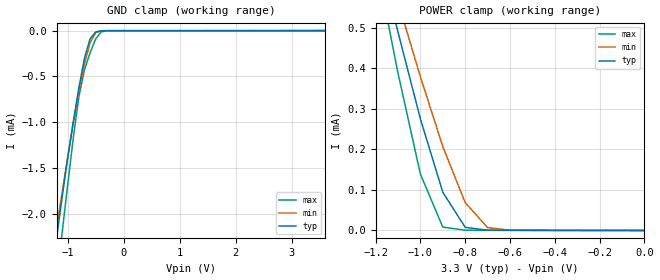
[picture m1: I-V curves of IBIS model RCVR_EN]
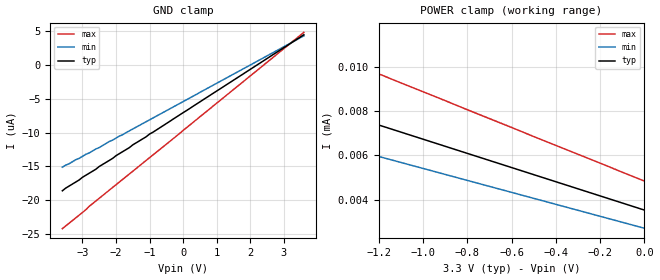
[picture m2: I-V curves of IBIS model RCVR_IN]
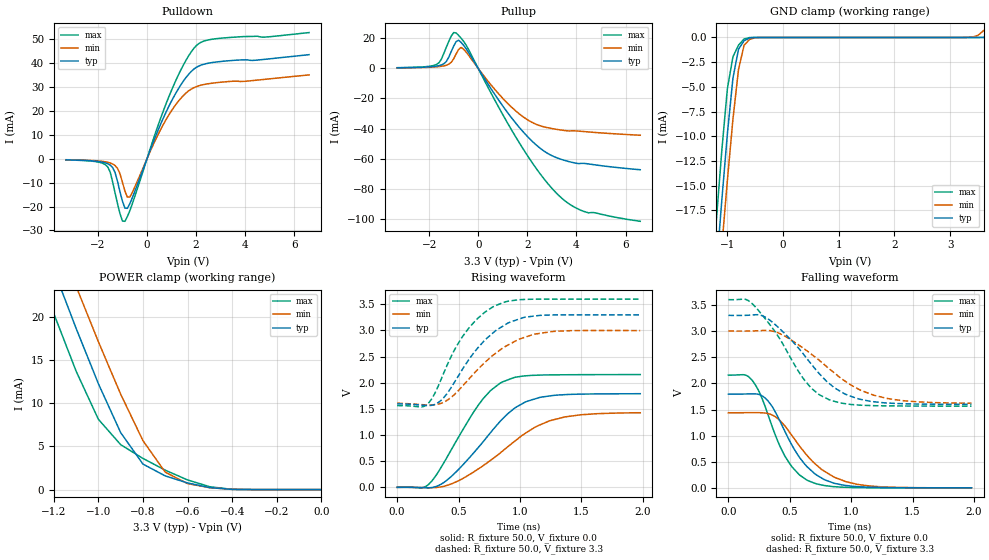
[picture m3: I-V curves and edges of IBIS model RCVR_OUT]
|   Texas Instruments Incorporated
|   Data Transmissions Products
|   IBIS Model for SN65MLVD2
|   8DRB SON Package
[IBIS Ver]   3.2
[Comment char]   |_char
[File name]   mlvd2.ibs
[File Rev]   1.0
[Date]   13Oct06
[Source]   File originated at Texas Instruments Incorporated.
   Data Transmission Products Group. All data based on
   Simulation Measurements.
[Notes]
[Disclaimer]
(C) Copyright Texas Instruments Incorporated 2006
   All rights reserved
  Texas Instruments Incorporated hereby grants the user of this IBIS
model a non-exclusive, nontransferable license to use this IBIS model
under the following terms.  Before using this IBIS model, the user
should read this license.  If the user does not accept these terms,
the IBIS model should be returned to Texas Instruments within 30 days.
  The user is granted this license only to use the IBIS model and
is not granted rights to sell, load, rent, lease or license the IBIS
model in whole or in part, or in modified form to anyone other than
user.  User may modify the IBIS model to suit its specific applications
but rights to derivative works and such modifications shall belong to
Texas Instruments.
  This IBIS model is provided on an "AS IS" basis and Texas Instruments
makes absolutely no warranty with respect to the information contained
herein.  TEXAS INSTRUMENTS DISCLAIMS AND CUSTOMER WAIVES ALL WARRANTIES,
EXPRESS OR IMPLIED, INCLUDING WARRANTIES OF MERCHANTABILITY OR FITNESS
FOR A PARTICULAR PURPOSE. The entire risk as to quality and performance
is with the Customer. ACCORDINGLY, IN NO EVENT SHALL THE COMPANY BE LIABLE
FOR ANY DAMAGES, WHETHER IN CONTRACT OR TORT,INCLUDING ANY LOST PROFITS
OR OTHER INCIDENTAL, CONSEQUENTIAL, EXEMPLARY, OR PUNITIVE DAMAGES ARISING
OUT OF THE USE OR APPLICATION OF THE IBIS model provided in this package.
Further, Texas Instruments reserves the right to discontinue or make changes
without notice to any product herein to improve reliability, function, or
design. Texas Instruments does not convey any license under patent rights
or any other intellectual property rights, including those of third parties.
Contact Texas Instruments at ATTN:DATA TRANSMISSIONS
[Copyright]   Copyright 2006, Texas Instruments, All Rights Reserved
[Component]   SN65MLVD2DRB
[Manufacturer]  Texas Instruments Incorporated
[Package]
|   typ   min   max
R_pkg   0.053   0.044   0.064
L_pkg   0.601nH   0.516nH   0.705nH
C_pkg   0.124pF   0.052pF   0.199pF
[Pin]   signal_name   model_name   R_pin   L_pin   C_pin
1   VCC   POWER   0.044   0.517n   0.192p
2   REBAR   RCVR_EN   0.064   0.705n   0.054p
3   R   RCVR_OUT   0.063   0.687n   0.054p
4   GND   GND   0.045   0.536n   0.199p
5   GND   GND   0.044   0.518n   0.196p
6   A   RCVR_IN   0.062   0.663n   0.052p
7   B   RCVR_IN   0.062   0.666n   0.053p
8   VCC   POWER   0.044   0.516n   0.194p
[Diff_pin]   inv_pin   vdiff   tdelay_typ   tdelay_min   tdelay_max
| The 'A' pin is Diff_pin and the 'B' pin is the inv_pin
   6   7   0.035   0   0   0
| Models and submodels in the file (3): RCVR_EN (Input), RCVR_IN (Input), RCVR_OUT (3-state)
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|   Receiver Enable Model
[Model]   RCVR_EN
Model_type   Input
|Signals   REBAR
Vinh = 2.0
Vinl = 0.8
|   typ   min   max
C_comp   4.10pF   3.83pF   4.30pF
|   typ   min   max
[Temperature Range]   25.0   85   -40
[Voltage range]   3.3V   3.0V   3.6V
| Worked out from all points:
|   GND clamp passes 1 mA (typ) near -0.90 V on its own axis
|   POWER clamp passes 1 mA (typ) near -1.32 V on its own axis
[GND_clamp]
|   Voltage   I(typ)   I(min)   I(max)
-3.6V     -16.3mA    -13.4mA    -20.8mA
-1.3V     -2.75mA    -2.57mA    -3.33mA
-1.2V     -2.27mA    -2.16mA    -2.76mA
-1.1V     -1.82mA    -1.77mA    -2.21mA
-900mV    -991uA     -1.01mA    -1.17mA
-800mV    -621uA     -665uA     -719uA
-700mV    -298uA     -359uA     -427uA
-600mV    -87.7uA    -132uA     -240uA
-500mV    -14.9uA    -21uA      -90.2uA
-400mV    -1.52uA    -1.46uA    -12.8uA
-300mV    -611nA     -376nA     -1.4uA
3.6V      162nA      525nA      103pA
[Power_clamp]
| Note that the[POWER_clamp]voltage table is referenced to Vcc
| and is calculated using Vtable=Vcc - Vmeasured.
|   Voltage   I(typ)   I(min)   I(max)
-3.3V     5.83mA     5.06mA     7.13mA
-1.2V     714uA      756uA      668uA
-1.1V     489uA      564uA      388uA
-1V       275uA      379uA      139uA
-900mV    94.4uA     207uA      8.25uA
-800mV    7.83uA     68.7uA     748nA
-700mV    564nA      7.16uA     602nA
-600mV    340nA      525nA      513nA
0V        64.4pA     58.2pA     103pA
|   Receiver Input Model
[Model]   RCVR_IN
Model_type   Input
| Signals   A.B
Vinl = 0.8V
Vinh = 1.2V
| variable   typ   min   max
C_comp   3.92pF   3.72pF   4.25pF
|   typ   min   max
[Temperature Range]   25.0   85   -40
[Voltage range]   3.3V   3.0V   3.6V
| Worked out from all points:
|   POWER clamp passes 1 mA (typ) near -3.06 V on its own axis
[GND_clamp]
|   Voltage   I(typ)   I(min)   I(max)
-3.6V     -18.6uA    -15.1uA    -24.2uA
-3.5V     -18.2uA    -14.8uA    -23.8uA
-2.5V     -15uA      -12.2uA    -19.7uA
3.6V      4.49uA     4.33uA     4.84uA
[Power_clamp]
| Note that the[POWER_clamp]voltage table is referenced to Vcc
| and is calculated using Vtable=Vcc - Vmeasured.
|   Voltage   I(typ)   I(min)   I(max)
-3.3V     7.92mA     1.68mA     31.7mA
-2.5V     193uA      32.1uA     566uA
-2.4V     91.4uA     11.2uA     388uA
-2.3V     26.7uA     9.01uA     222uA
-2.2V     11.2uA     8.66uA     87.4uA
-2.1V     10.3uA     8.38uA     18.8uA
-2V       9.93uA     8.11uA     12.9uA
-1.7V     8.97uA     7.3uA      11.7uA
-1.6V     8.65uA     7.03uA     11.3uA
0V        3.53uA     2.71uA     4.84uA
|   Receiver Output Model
[Model]   RCVR_OUT
Model_type   3-state
| Signals   R
Vmeas = 1.65V   |Reference voltage for timing measurements
Cref = 15pF   |Timing specification test load capacitance value
Vref = 0   |Timing specification test load voltage; GND
| variable   typ   min   max
C_comp   4.13pF   3.88pF   4.46pF
|   typ   min   max
[Temperature Range]   25.0   85   -40
[Voltage range]   3.3V   3.0V   3.6V
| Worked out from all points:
|   slope of the pulldown table from 0 to 0.495 V, typ, clamps not added: 38 ohm
|   slope of the pullup table from 0 to 0.495 V, typ, clamps not added: 38.6 ohm
|   GND clamp passes 1 mA (typ) near -0.78 V on its own axis
|   POWER clamp passes 1 mA (typ) near -0.63 V on its own axis
|   rising waveform, R_fixture 50.0, V_fixture 0.0: 20-80 % time 407ps typ, 499ps min, 341ps max; typ from 0 V to 1.79 V
|   falling waveform, R_fixture 50.0, V_fixture 0.0: 20-80 % time 276ps typ, 332ps min, 238ps max; typ from 1.79 V to 0.003 V
|   rising waveform, R_fixture 50.0, V_fixture 3.3: 20-80 % time 336ps typ, 389ps min, 299ps max; typ from 1.59 V to 3.3 V
|   falling waveform, R_fixture 50.0, V_fixture 3.3: 20-80 % time 395ps typ, 475ps min, 338ps max; typ from 3.3 V to 1.6 V
[Pulldown]
|   Voltage   I(typ)   I(min)   I(max)
-3.3V     -470uA     -410uA     -490uA
-1.6V     -2.085mA   -1.492mA   -3.417mA
-1.4V     -3.695mA   -2.193mA   -9.687mA
-1.2V     -9.523mA   -4.041mA   -18.86mA
-1V       -17.78mA   -9.855mA   -26.09mA
-900mV    -20.64mA   -13.51mA   -26.18mA
-700mV    -18.83mA   -16.02mA   -21.77mA
900mV     22.14mA    18.5mA     26.2mA
1.5V      32.76mA    26.63mA    39.57mA
2V        38.19mA    30.14mA    47.24mA
2.8V      40.46mA    31.8mA     50.21mA
6.6V      43.55mA    35.08mA    52.8mA
[Pullup]
|   Voltage   I(typ)   I(min)   I(max)
| Note that the[Pullup]voltage table is referenced to Vcc
| and is calculated using Vtable=Vcc - Vmeasured.
-3.3V     440uA      360uA      490uA
-1.7V     1.542mA    1.06mA     2.62mA
-1.3V     4.581mA    2.12mA     14.07mA
-1V       14.87mA    6.366mA    23.86mA
-900mV    17.81mA    9.615mA    23.62mA
-600mV    15.47mA    12.91mA    18.13mA
800mV     -20.28mA   -16.29mA   -24.81mA
1.8V      -41.63mA   -31.82mA   -52.78mA
2.5V      -52.79mA   -38.03mA   -69.62mA
3.2V      -59.43mA   -40.55mA   -83.19mA
4.3V      -63.16mA   -41.99mA   -95.12mA
6.6V      -67.4mA    -44.44mA   -101.7mA
[GND_clamp]
|   Voltage   I(typ)   I(min)   I(max)
| Outputs in High Impedance (off)
-3.6V     -212.1mA   -209.7mA   -214.2mA
-1.2V     -23.65mA   -28.19mA   -18.68mA
-1.1V     -16.49mA   -21.21mA   -11.44mA
-1V       -9.758mA   -14.48mA   -5.194mA
-900mV    -4.108mA   -8.262mA   -1.954mA
-800mV    -1.191mA   -3.239mA   -779.7uA
-700mV    -331.4uA   -789.1uA   -157.8uA
-600mV    -38.04uA   -194.3uA   -10.33uA
-500mV    -1.877uA   -29.93uA   -245.4nA
3.3V      74.32pA    2.978uA    70.8pA
3.5V      44.42nA    218.9uA    77.09pA
3.6V      1.392uA    698uA      81.14pA
[POWER_clamp]
|   Voltage   I(typ)   I(min)   I(max)
| Note that the [POWER_clamp] voltage table is referenced to Vcc
| and is calculated using Vtable = Vcc - Vmeasured.
| Outputs in Tri-state.
-3.3V     177.5mA    176.8mA    177.7mA
-1.3V     32.31mA    36.82mA    27.39mA
-1.2V     25.4mA     30.11mA    20.36mA
-1.1V     18.66mA    23.52mA    13.71mA
-1V       12.25mA    17.11mA    8.134mA
-900mV    6.595mA    11.04mA    5.201mA
-800mV    2.952mA    5.665mA    3.608mA
-700mV    1.584mA    2.016mA    2.249mA
-600mV    771.1uA    698uA      1.12mA
-500mV    232uA      218.9uA    331.8uA
-400mV    27.19uA    35.23uA    29.9uA
0V        74.32pA    76.81pA    81.14pA
[Ramp]
|   typ   min   max
dV/dt_r   1.076V/407ps   0.862V/501ps   1.294V/342ps
dV/dt_f   1.022V/396ps   0.832V/479ps   1.222V/338ps
R_load = 50
[Rising Waveform]
R_fixture = 50.0
V_fixture = 0.0
C_fixture = 0p
L_fixture = 0n
|   V(typ)   V(min)   V(max)
0s        0V         0V         0V
200ps     -5mV       -4mV       -9mV
260ps     -9mV       -8mV       65mV
400ps     127mV      33mV       550mV
660ps     760mV      351mV      1.569V
860ps     1.312V     697mV      2.017V
1.04ns    1.627V     1.028V     2.131V
1.24ns    1.746V     1.271V     2.149V
1.5ns     1.782V     1.388V     2.154V
1.98ns    1.79V      1.426V     2.156V
[Falling Waveform]
R_fixture = 50.0
V_fixture = 0.0
C_fixture = 0p
L_fixture = 0n
|   V(typ)   V(min)   V(max)
0s        1.794V     1.437V     2.158V
160ps     1.798V     1.44V      2.135V
240ps     1.794V     1.441V     1.889V
300ps     1.718V     1.433V     1.555V
360ps     1.547V     1.392V     1.151V
460ps     1.084V     1.187V     610mV
640ps     408mV      624mV      151mV
860ps     92mV       210mV      26mV
1.06ns    25mV       66mV       8mV
1.98ns    3mV        3mV        3mV
[Rising Waveform]
R_fixture = 50.0
V_fixture = 3.3
V_fixture_min = 3.0
V_fixture_max = 3.6
C_fixture = 0p
L_fixture = 0n
|   V(typ)   V(min)   V(max)
0s        1.595V     1.609V     1.563V
200ps     1.571V     1.581V     1.537V
260ps     1.563V     1.574V     1.624V
380ps     1.717V     1.63V      2.19V
520ps     2.213V     1.904V     2.84V
640ps     2.619V     2.214V     3.193V
800ps     2.992V     2.559V     3.474V
920ps     3.159V     2.742V     3.563V
1.12ns    3.276V     2.929V     3.597V
1.98ns    3.297V     2.997V     3.598V
[Falling Waveform]
R_fixture = 50.0
V_fixture = 3.3
V_fixture_min = 3.0
V_fixture_max = 3.6
C_fixture = 0p
L_fixture = 0n
|   V(typ)   V(min)   V(max)
0s        3.3V       3V         3.6V
160ps     3.302V     3V         3.585V
320ps     3.237V     3.012V     3.176V
440ps     2.995V     2.928V     2.767V
620ps     2.533V     2.655V     2.062V
820ps     2V         2.281V     1.688V
960ps     1.786V     2.027V     1.609V
1.2ns     1.645V     1.764V     1.573V
1.48ns    1.608V     1.658V     1.567V
1.98ns    1.599V     1.621V     1.566V
